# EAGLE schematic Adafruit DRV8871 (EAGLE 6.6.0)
COMPANY: ADAFRUIT INDUSTRIES; DRAWN: KTOWN; REV: A
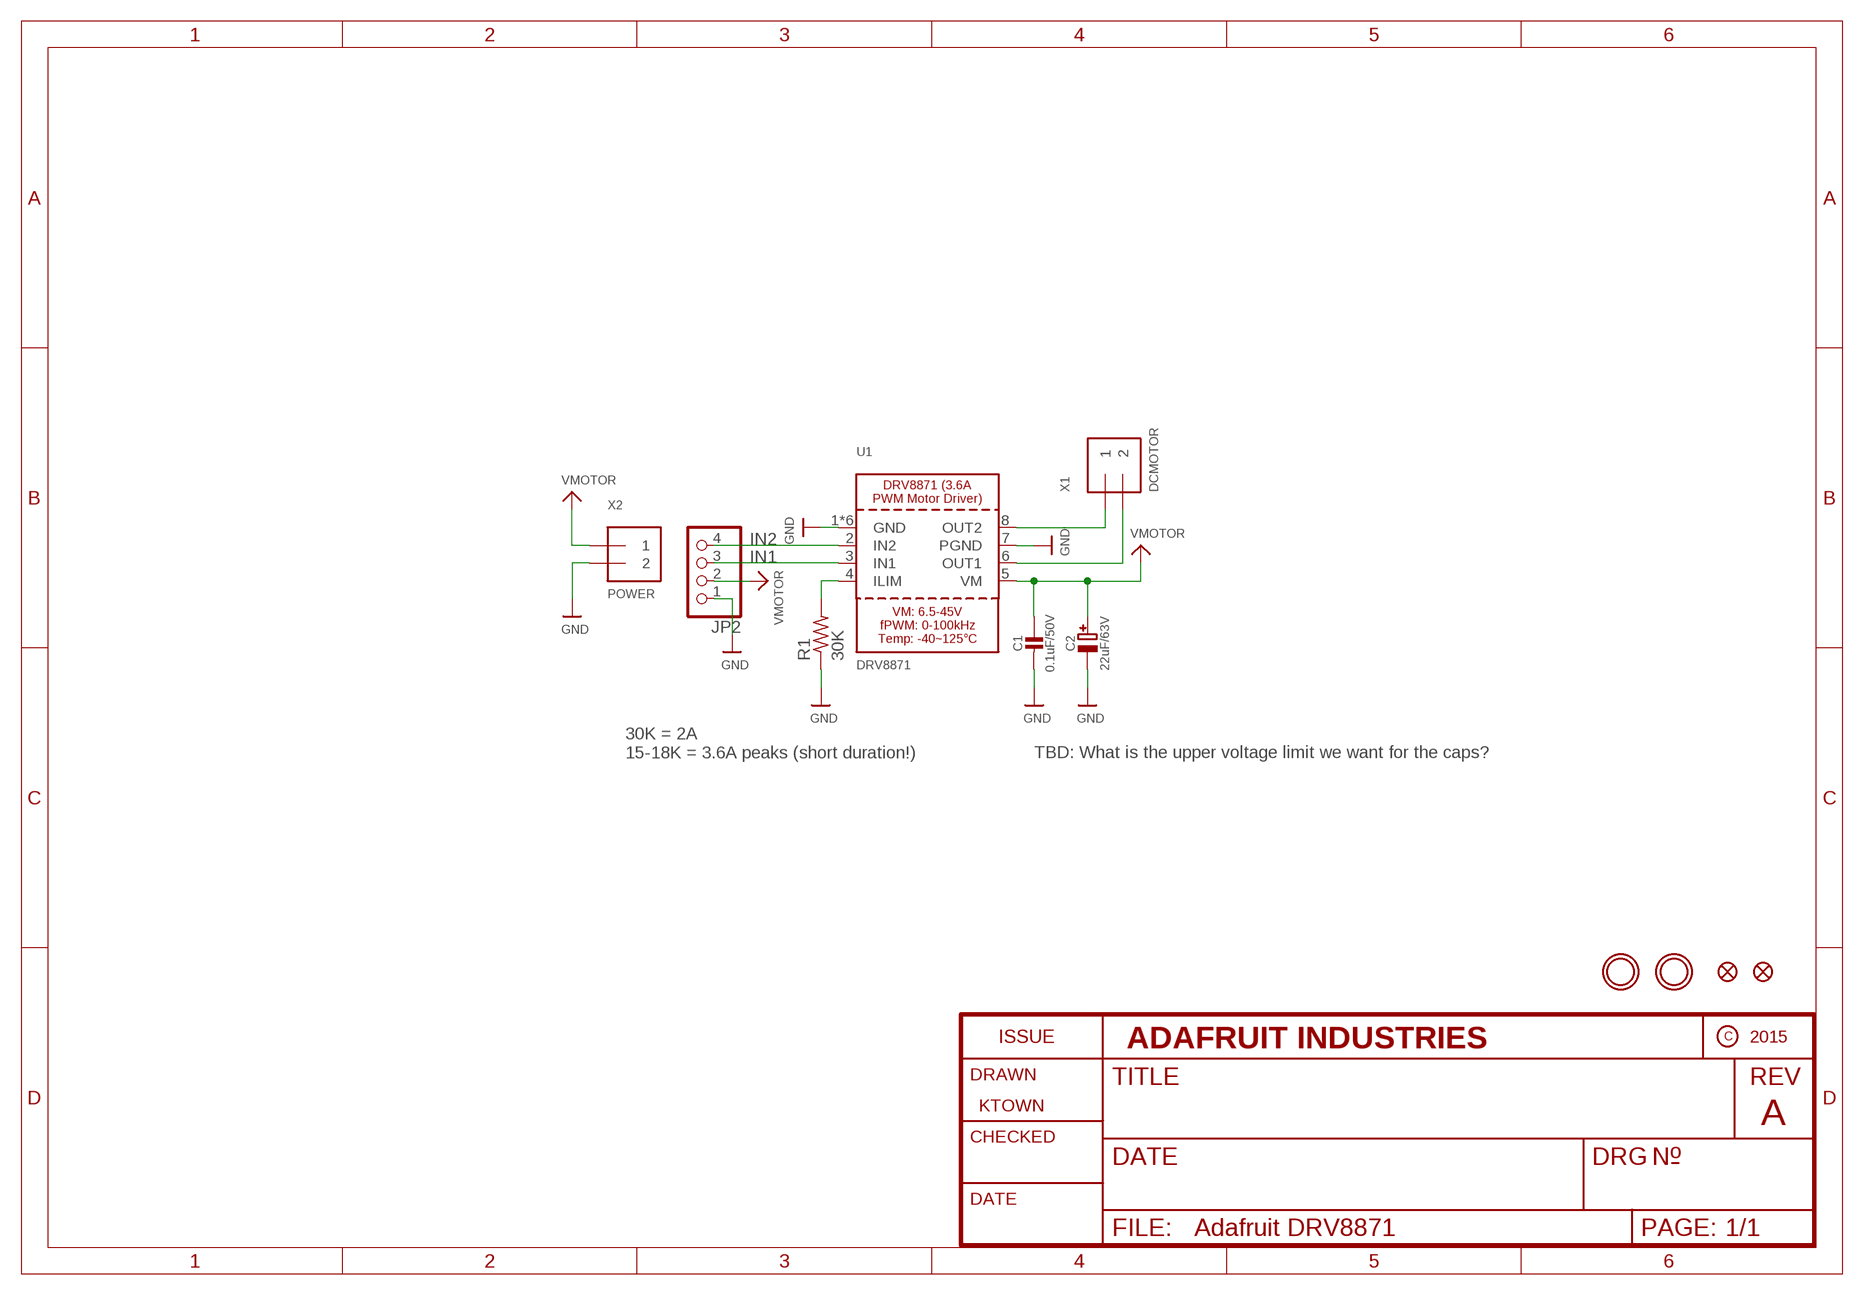
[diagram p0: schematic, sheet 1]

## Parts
C1  0.1uF/50V  CAP_CERAMIC0805-NOOUTLINE  [0805-NO]
C2  22uF/63V  CAP_ELECTROLYTICPANASONIC_D  [PANASONIC_D]
FID1  FIDUCIAL""  [FIDUCIAL_1MM]
FID2  FIDUCIAL""  [FIDUCIAL_1MM]
JP2  HEADER-1X476MIL  [1X04_ROUND_76]
R1  30K  FLIPFLOP-RES  [0805-THM]
U1  DRV8871  [HSOP8]
U$9  MOUNTINGHOLE2.5  [MOUNTINGHOLE_2.5_PLATED]
U$10  MOUNTINGHOLE2.5  [MOUNTINGHOLE_2.5_PLATED]
X1  DCMOTOR  TERMBLOCK_1X2  [TERMBLOCK_1X2-3.5MM]
X2  POWER  TERMBLOCK_1X2  [TERMBLOCK_1X2-3.5MM]

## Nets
GND: C1.2 C2.- JP2.1 R1.1 U1.1(GND) U1.7(PGND) U1.GND U1.P$1(GND) U1.P$2(GND) U1.P$3(GND) U1.P$4(GND) X2.2
IN1: JP2.3 U1.3(IN1)
IN2: JP2.4 U1.2(IN2)
N$1: R1.2 U1.4(ILIM)
OUT1: U1.6(OUT1) X1.2
OUT2: U1.8(OUT2) X1.1
VMOTOR: C1.1 C2.+ JP2.2 U1.5(VM) X2.1

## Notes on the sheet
- 30K = 2A
  15-18K = 3.6A peaks (short duration!)
- TBD: What is the upper voltage limit we want for the caps?

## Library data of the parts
C1 = microbuilder:CAP_CERAMIC: Ceramic Capacitors
C2 = microbuilder:CAP_ELECTROLYTIC: Electrolytic Capacitors
FID1 FID2 = microbuilder:FIDUCIAL: Fiducial Alignment Points; BOM: EXCLUDE
JP2 = microbuilder:HEADER-1X4: PIN HEADER
R1 = adafruit:FLIPFLOP-RES: Flip Flop resistor
U1 = microbuilder:DRV8871: DRV8871 - 3.6A PWM Motor Driver
U$9 U$10 = microbuilder:MOUNTINGHOLE: Mounting Hole; BOM: EXCLUDE
X1 X2 = microbuilder:TERMBLOCK_1X2: 3.5mm Terminal block

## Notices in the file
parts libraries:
microbuilder: This work is placed in the public domain, and may be freely used for commercial and non-commercial work with the following conditions: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
